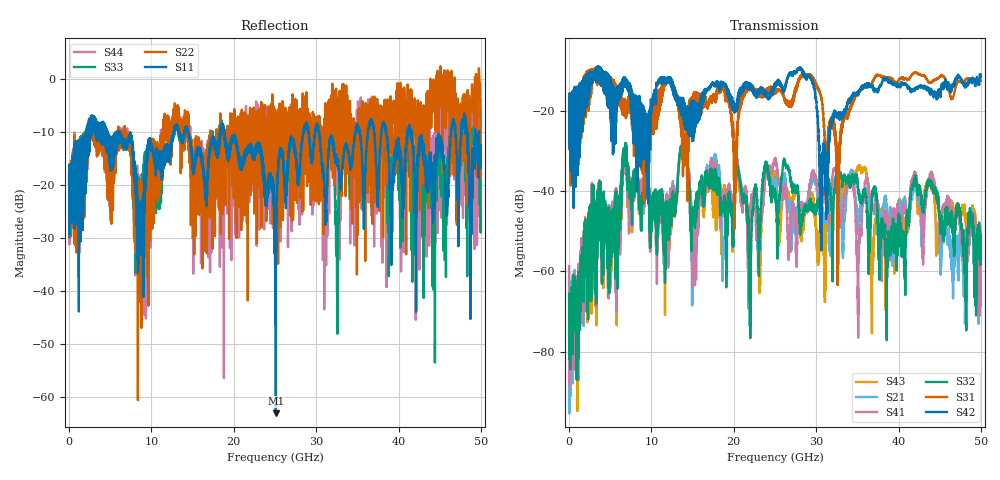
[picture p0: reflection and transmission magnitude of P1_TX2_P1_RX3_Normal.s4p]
!Keysight Technologies,N5225B,MY57041031,A.13.20.10
!Date: Friday, May 31, 2019 11:17:12
!Correction: S11(Full 4 Port(1,2,3,4))
!S12(Full 4 Port(1,2,3,4))
!S13(Full 4 Port(1,2,3,4))
!S14(Full 4 Port(1,2,3,4))
!S21(Full 4 Port(1,2,3,4))
!S22(Full 4 Port(1,2,3,4))
!S23(Full 4 Port(1,2,3,4))
!S24(Full 4 Port(1,2,3,4))
!S31(Full 4 Port(1,2,3,4))
!S32(Full 4 Port(1,2,3,4))
!S33(Full 4 Port(1,2,3,4))
!S34(Full 4 Port(1,2,3,4))
!S41(Full 4 Port(1,2,3,4))
!S42(Full 4 Port(1,2,3,4))
!S43(Full 4 Port(1,2,3,4))
!S44(Full 4 Port(1,2,3,4))
!S4P File: Measurements: <S11,S12,S13,S14>,
!<S21,S22,S23,S24>,
!<S31,S32,S33,S34>,
!<S41,S42,S43,S44>:
# Hz S  dB  R 50.0
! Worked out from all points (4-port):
!   5000 points, 10 MHz to 50 GHz, reference 50 ohm
!   strongest paths, dB at 10 MHz, 12.51 GHz, 25.01 GHz, 37.51 GHz, 50 GHz:
!     S42: -19.6, -14.4, -13.6, -14.9, -11.1
!     S31: -19.5, -13.0, -15.4, -11.1, -12.5
!     S32: -65.6, -42.5, -41.4, -51.1, -53.0
!     S41: -58.7, -40.0, -32.4, -43.9, -62.3
!     S21: -60.1, -39.5, -37.9, -48.4, -58.4
!     S43: -62.2, -43.3, -35.9, -46.6, -52.5
!   lowest |S11| = -63.1 dB at 25.1 GHz (marker M1), VSWR 1.00, Z = 49.9 - j0.032 ohm
!   |S11| at or under -10 dB: 6.091 GHz to 12.71 GHz (6.616 GHz wide, 70.4 % of centre); 18.82 GHz to 28.43 GHz (9.605 GHz wide, 40.7 % of centre); 41.58 GHz to 46.39 GHz (4.81 GHz wide, 10.9 % of centre)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
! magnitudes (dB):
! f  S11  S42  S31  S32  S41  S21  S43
! 10 MHz  -19.8  -19.6  -19.5  -65.6  -58.7  -60.1  -62.2
! 6.75 GHz  -12.6  -13.5  -20.8  -30.3  -31.4  -31.3  -30.6
! 13.99 GHz  -10.2  -21.1  -31.1  -29.5  -30.3  -29.2  -30.5
! 15.18 GHz  -16.8  -17.9  -22.8  -46.1  -55.5  -53.1  -48.4
! 25.1 GHz  -63.1  -13.7  -15.1  -41.9  -32.6  -37.9  -36.5
! 30.63 GHz  -14.8  -40.5  -17.0  -41.7  -42.2  -42.3  -48.7
! 50 GHz  -12.6  -11.1  -12.5  -53.0  -62.3  -58.4  -52.5
